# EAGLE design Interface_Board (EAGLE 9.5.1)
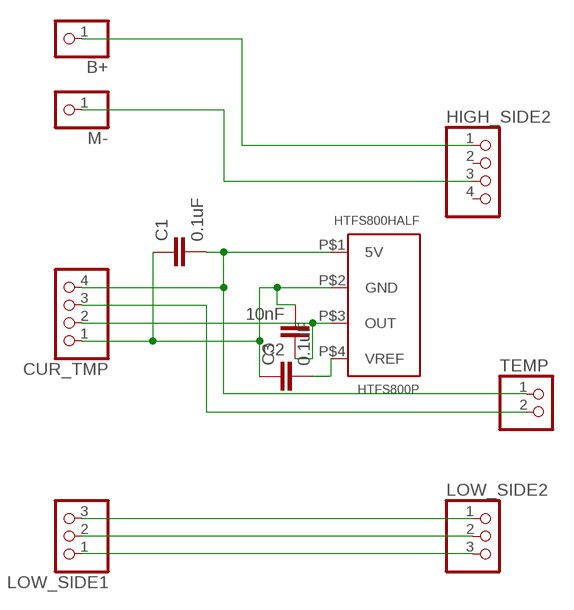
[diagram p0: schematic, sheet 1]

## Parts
B+  PINHD-1X1  [1X01]
C1  0.1uF  C-EUC1206  [C1206]
C2  10nF  C-EUC1206  [C1206]
C3  0.1uF  C-EUC1206  [C1206]
CUR_TMP  PINHD-1X4  [1X04]
HIGH_SIDE2  PINHD-1X4  [1X04]
HTFS800P  HTFS800HALF  [HTFS800-HALF]
LOW_SIDE1  PINHD-1X3  [1X03]
LOW_SIDE2  PINHD-1X3  [1X03]
M-  PINHD-1X1  [1X01]
TEMP  PINHD-1X2  [1X02]

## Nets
GND: LOW_SIDE1.2 LOW_SIDE2.2
N$1: C1.1 C2.2 C3.1 CUR_TMP.1 HTFS800P.P$2(GND)
N$2: C2.1 CUR_TMP.2 HTFS800P.P$3(OUT)
N$3: HIGH_SIDE2.3 M-.1
N$4: C1.2 CUR_TMP.4 HTFS800P.P$1(5V) TEMP.1
N$5: CUR_TMP.3 TEMP.2
N$7: LOW_SIDE1.3 LOW_SIDE2.1
N$8: B+.1 HIGH_SIDE2.1
N$9: C3.2 HTFS800P.P$4(VREF)
N$11: LOW_SIDE1.1 LOW_SIDE2.3
Unconnected: HIGH_SIDE2.2 HIGH_SIDE2.4

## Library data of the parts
B+ M- = pinhead:PINHD-1X1: PIN HEADER
C1-C3 = resistor:C-EU: CAPACITOR, European symbol
CUR_TMP HIGH_SIDE2 = pinhead:PINHD-1X4: PIN HEADER
HTFS800P = Ians parts:HTFS800
LOW_SIDE1 LOW_SIDE2 = pinhead:PINHD-1X3: PIN HEADER
TEMP = pinhead:PINHD-1X2: PIN HEADER

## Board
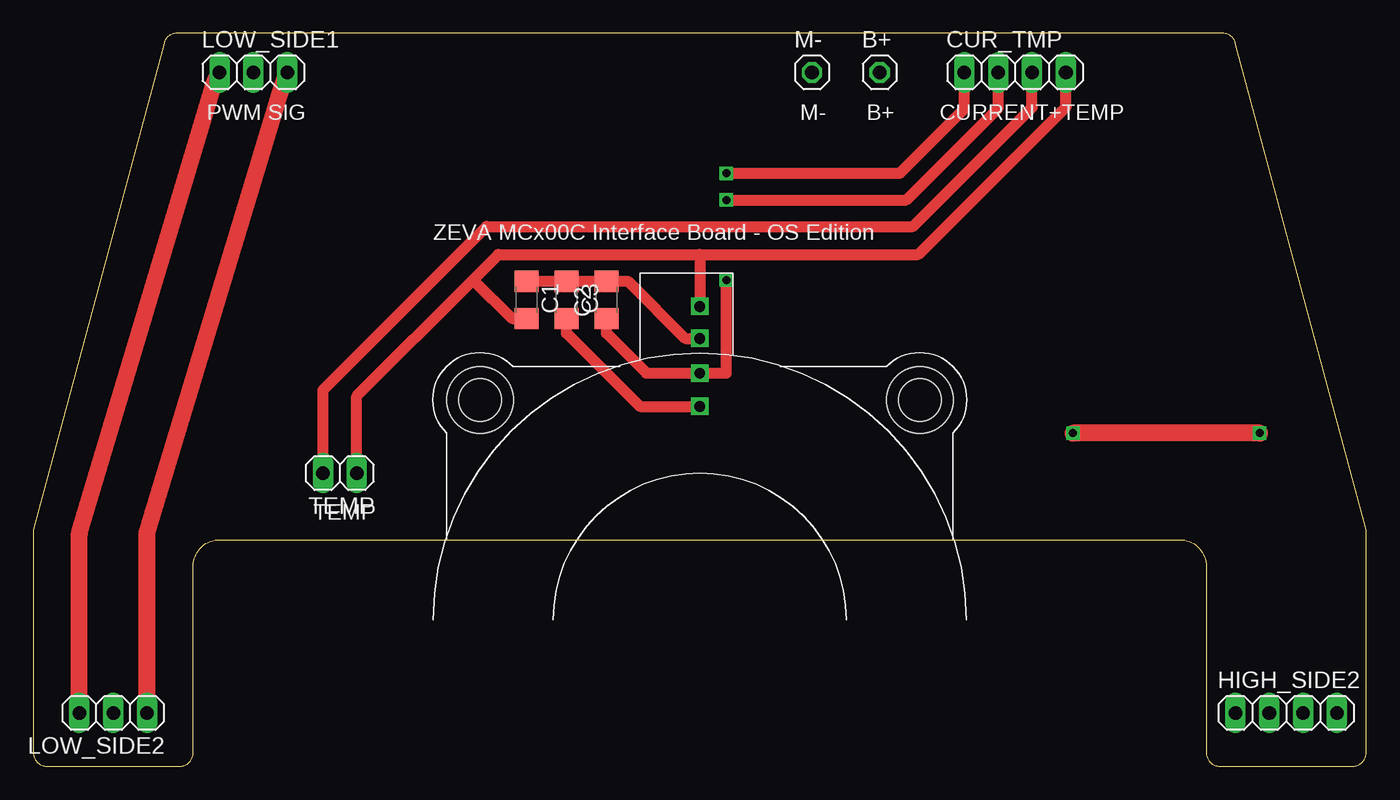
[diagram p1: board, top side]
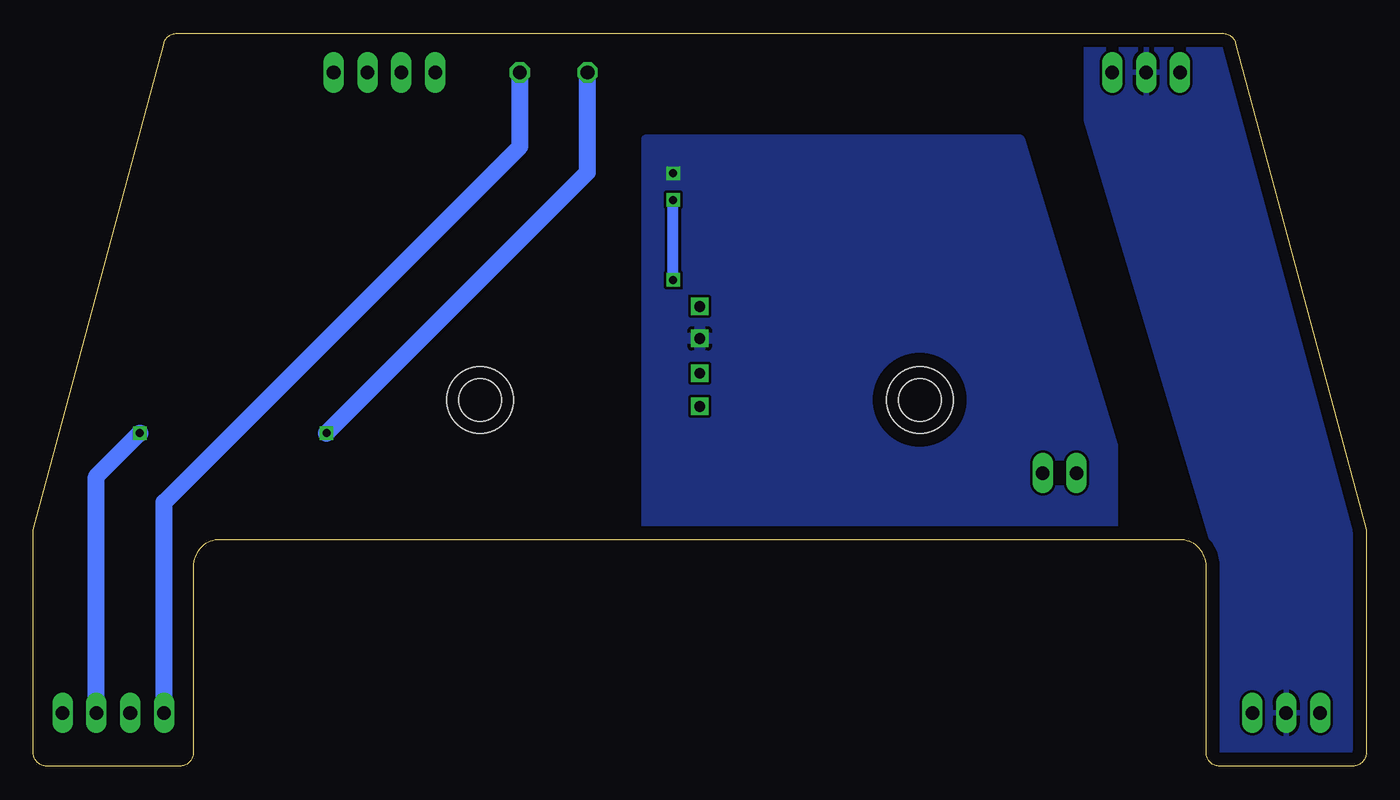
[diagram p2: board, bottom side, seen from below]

Size 100 x 55 mm. Coordinates in mm from the lower left corner, seen from the top.
Outline: 90.2,54.26 arc75 89.23,55 10.77,55 arc75 9.8,54.26 0,17.75 0,1 arc90 1,0 11,0 arc90 12,1 12,15 arc-90 14,17 86,17 arc-90 88,15 88,1 arc90 89,0 99,0 arc90 100,1 100,17.75 90.2,54.26
Copper layers (1*16): Top 0.035mm / dielectric 1.5mm / Bottom 0.035mm
Design rules "default": minimum track width 10mil, minimum drill 24mil, track to track 8mil, track to pad 8mil, pad to pad 8mil, via to via 8mil, smd to smd 8mil, copper to edge 40mil, drill to drill 8mil, minimum pad ring 10mil, minimum via ring 8mil, stop-mask expansion 4mil, vias tented up to drill 0mil, thermal gap 10mil
Holes 5 mm at 33.5,27.5 66.5,27.5

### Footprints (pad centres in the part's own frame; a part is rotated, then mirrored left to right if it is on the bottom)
1X01 = drill 1.016 octagon: 1 0,0
C1206 = smd 1.6 x 1.8: 1 -1.4,0; 2 1.4,0
1X04 = drill 1.016 long: 1 -3.81,0; 2 -1.27,0; 3 1.27,0; 4 3.81,0
HTFS800-HALF = drill 0.8 square: P$1 0,-23.5; P$2 0,-21.1; P$3 0,-18.5; P$4 0,-16 | hole 3.2: 16.5,-16.5; -16.5,-16.5
1X03 = drill 1.016 long: 1 -2.54,0; 2 0,0; 3 2.54,0
1X02 = drill 1.016 long: 1 -1.27,0; 2 1.27,0

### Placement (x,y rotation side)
B+  63.5,52.07 0 top
C1  37,35 270 top
C2  43,35 90 top
C3  40,35 270 top
CUR_TMP  73.66,52.07 0 top
HIGH_SIDE2  94,4 0 top
HTFS800P  50,11 180 top
LOW_SIDE1  16.51,52.07 0 top
LOW_SIDE2  6,4 180 top
M-  58.42,52.07 0 top
TEMP  23,22 180 top

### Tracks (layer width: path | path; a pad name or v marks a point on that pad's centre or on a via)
GND
  pour Bottom: 10,55 21,55 21,48.5 11,15 11,0 0,0 0,18
N$1  (via drill 0.6)
  Top 0.813: HTFS800P.P$2 48.9,32.1 44.6,36.4 C2.2 C3.1 C1.1 | CUR_TMP.1 69.85,49.35 65,44.5 v52,44.5
  pour Bottom: 26,47 54,47 54,16 19,16 19,24
N$2  (via drill 0.6)
  Top 0.813: v52,36.5 52,29.5 HTFS800P.P$3 46,29.5 43,32.5 C2.1 | CUR_TMP.2 72.39,49.39 65.5,42.5 v52,42.5
  Bottom 0.813: v52,36.5 v52,42.5
N$3  (via drill 0.6)
  Top 1.27: v92,25 v78,25
  Bottom 1.27: M-.1 58.42,44.58 v78,25 | v92,25 95.27,21.73 HIGH_SIDE2.3
N$4
  Top 0.813: TEMP.1 24.27,27.77 33,36.5 | 50,38.4 HTFS800P.P$1 | 33,36.5 34.9,38.4 50,38.4 | C1.2 35.9,33.6 33,36.5 | CUR_TMP.4 77.47,49.47 66.4,38.4 50,38.4
N$5
  Top 0.813: TEMP.2 21.73,28.23 34,40.5 66,40.5 74.93,49.43 CUR_TMP.3
N$7
  Top 1.27: LOW_SIDE2.1 8.54,17.54 18.5,50.5 LOW_SIDE1.3
N$8
  Bottom 1.27: B+.1 63.5,46.5 90.19,19.81 HIGH_SIDE2.1
N$9
  Top 0.813: HTFS800P.P$4 45.5,27 40,32.5 C3.2
N$11
  Top 1.27: LOW_SIDE2.3 3.46,17.46 13.5,51 LOW_SIDE1.1

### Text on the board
tPlace: PWM SIG | M- | B+ | CURRENT+TEMP | ZEVA MCx00C Interface Board - OS Edition | TEMP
